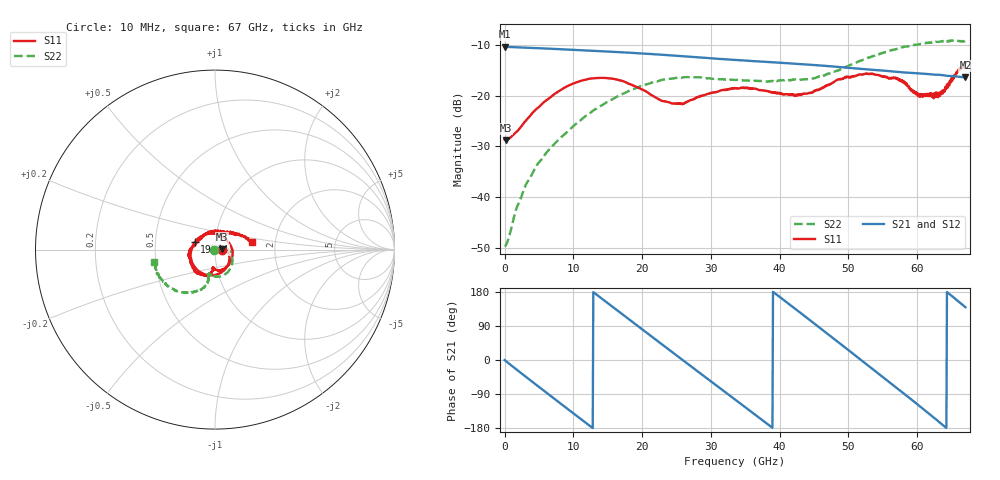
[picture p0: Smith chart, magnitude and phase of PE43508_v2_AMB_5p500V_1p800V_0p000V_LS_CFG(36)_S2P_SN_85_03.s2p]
!Keysight Technologies,N5227A,US51270237,A.10.43.00
!Date: Wednesday, August 22, 2018 17:10:19
!Correction: S11(Full 2 Port(1,3))
!S31(Full 2 Port(1,3))
!S13(Full 2 Port(1,3))
!S33(Full 2 Port(1,3))
!S2P File: Measurements: S11, S31, S13, S33:
# Hz S  dB  R 50
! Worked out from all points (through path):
!   801 points, 10 MHz to 67 GHz, reference 50 ohm
!   highest |S21| = -10.33 dB at 10 MHz (marker M1); lowest = -16.4 dB at 67 GHz (marker M2)
!   group delay of S21, straight-line fit = 38.7 ps
!   lowest |S11| = -28.8 dB at 261.2 MHz (marker M3), VSWR 1.08, Z = 53.8 + j0.078 ohm
!   |S11| at or under -10 dB: start of sweep to end of sweep
!   |S22| runs from -49.7 to -9.1 dB; largest |S21 - S12| = 0.0017
!   S11 on the Smith chart (normalised r, x): 10 MHz: 1.08, -0.00; 19.44 GHz: 0.79, +0.07; 67 GHz: 1.52, +0.13
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1e7  -28.63 -1.0  -10.33 -0.2  -10.33 -0.2  -49.68 -176.5
2.612125e8  -28.77 1.1  -10.36 -3.9  -10.36 -3.9  -49.24 156.3
1.852225e9  -26.99 4.8  -10.45 -26.7  -10.45 -26.7  -41.77 91.6
4.615562e9  -22.63 -11.9  -10.61 -65.6  -10.61 -65.6  -33.87 59.5
7.71385e9  -19.26 -46.6  -10.79 -108.9  -10.79 -108.8  -28.87 39.1
1.123082e10  -17.00 -89.6  -11.01 -157.7  -11.01 -157.7  -24.64 13.7
1.483154e10  -16.52 -135.4  -11.26 152.5  -11.26 152.5  -21.30 -9.6
1.94371e10  -18.38 159.1  -11.61 88.9  -11.61 88.9  -18.30 -38.2
2.236791e10  -20.66 108.6  -11.87 48.4  -11.86 48.4  -17.09 -55.8
2.571741e10  -21.54 40.5  -12.18 2.4  -12.19 2.4  -16.45 -73.9
2.722469e10  -20.82 11.6  -12.33 -18.3  -12.34 -18.3  -16.32 -80.8
3.049045e10  -19.29 -33.9  -12.66 -63.0  -12.66 -63.0  -16.67 -93.2
3.3505e10  -18.53 -63.9  -12.93 -104.2  -12.94 -104.2  -16.88 -99.8
3.903168e10  -19.28 -94.8  -13.40 179.8  -13.41 180.0  -17.07 -104.1
4.472582e10  -19.36 -95.2  -13.90 100.4  -13.89 100.5  -16.62 -104.4
4.740542e10  -17.67 -99.5  -14.20 62.7  -14.19 62.7  -15.52 -103.2
5.058745e10  -16.13 -113.1  -14.55 17.8  -14.54 17.8  -13.79 -104.2
5.586291e10  -16.62 -156.8  -15.12 -57.2  -15.11 -57.5  -11.15 -120.1
5.787261e10  -17.34 -179.3  -15.38 -86.1  -15.38 -86.3  -10.44 -127.8
6.021726e10  -19.65 145.2  -15.58 -119.8  -15.58 -120.1  -9.84 -137.1
6.272939e10  -19.34 89.0  -15.85 -156.6  -15.86 -156.9  -9.37 -148.6
6.7e10  -13.48 10.8  -16.39 139.3  -16.46 139.2  -9.22 -168.6
